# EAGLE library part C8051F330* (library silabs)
8kB ILP Flash MCU Family Source: www.silabs.com .. C8051F33x.pdf
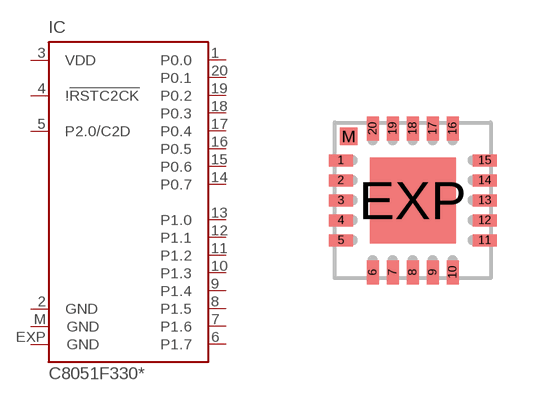
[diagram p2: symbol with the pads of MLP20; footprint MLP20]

Designator prefix IC

## C8051F330/1 (MPN: C8051F330-GM; OC_FARNELL: 1291513; OC_NEWARK: 24M1242)  [MLP20]
1  P0.0
2  GND  pwr
3  VDD  pwr
4  !!RSTC2CK  in
5  P2.0/C2D
6  P1.7
7  P1.6
8  P1.5
9  P1.4
10  P1.3
11  P1.2
12  P1.1
13  P1.0
14  P0.7
15  P0.6
16  P0.5
17  P0.4
18  P0.3
19  P0.2
20  P0.1
EXP  GND  pwr
M  GND  pwr

## Footprint MLP20 (pad centres in mm)
MLP 20 Source: www.silabs.com .. C8051F33x.pdf
smd 0.6 x 0.3: 1 -1.8,1; 2 -1.8,0.5; 3 -1.8,0; 4 -1.8,-0.5; 5 -1.8,-1; 11 1.8,-1; 12 1.8,-0.5; 13 1.8,0; 14 1.8,0.5; 15 1.8,1
smd 0.3 x 0.6: 6 -1,-1.8; 7 -0.5,-1.8; 8 0,-1.8; 9 0.5,-1.8; 10 1,-1.8; 16 1,1.8; 17 0.5,1.8; 18 0,1.8; 19 -0.5,1.8; 20 -1,1.8
smd 2.15 x 2.15: EXP 0,0
smd 0.435 x 0.435: M -1.6,1.6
